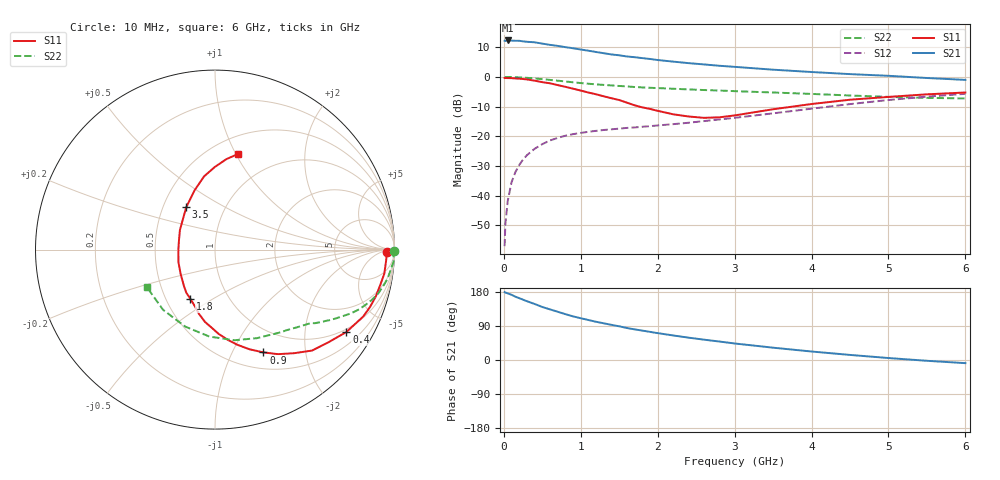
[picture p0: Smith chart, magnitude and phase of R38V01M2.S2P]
! SIEMENS Small Signal Semiconductors
! BFR181
! Si NPN RF Bipolar Junction Transistor in SOT23
! VCE = 8 V  IC = 1.2 mA
! Common Emitter S-Parameters:  May  1996
# GHz  S  MA  R  50
!  f  S11  S21  S12  S22
! GHz  MAG  ANG  MAG  ANG  MAG  ANG  MAG  ANG
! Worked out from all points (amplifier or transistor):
!   36 points, 10 MHz to 6 GHz, reference 50 ohm
!   highest |S21| = 12.3 dB at 50 MHz (marker M1)
!   |S21| within 3 dB of that: start of sweep to 987.8 MHz
!   unconditionally stable (mu >= 1): 1.967 GHz to 3.654 GHz
!   at 250 MHz: K = 0.17, MSG = 19.9 dB, |S12| = -27.9 dB
!   at 1.4 GHz: K = 0.80, MSG = 12.6 dB, |S12| = -17.7 dB
!   at 6 GHz: K = 0.86, MSG = 2.4 dB, |S12| = -5.7 dB
!   S11 on the Smith chart (normalised r, x): 10 MHz: 42, -14; 400 MHz: 0.90, -3.25; 900 MHz: 0.70, -1.33; 1.8 GHz: 0.66, -0.40; 3.5 GHz: 0.66, +0.34; 6 GHz: 0.67, +1.01
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0.01  0.9582 -0.8  4.069 179.2  0.0014 97.4  0.9984 -0.4
0.02  0.9573 -1.6  4.023 178.0  0.0033 92.5  0.9906 -0.8
0.05  0.9551 -3.9  4.115 175.9  0.008 87.2  0.9955 -2.0
0.1  0.9528 -8.1  4.088 172.1  0.0167 84.5  0.9968 -3.9
0.15  0.9415 -12.1  4.066 167.1  0.0248 81.3  0.9876 -5.9
0.2  0.9331 -16.3  4.062 163.2  0.0327 78.9  0.9808 -7.8
0.3  0.9061 -24.3  3.907 155.1  0.0479 75.0  0.9642 -11.4
0.4  0.8641 -32.1  3.832 147.9  0.0614 70.2  0.9432 -14.8
0.5  0.8153 -39.4  3.642 139.9  0.0735 66.1  0.9156 -18.0
0.6  0.7804 -46.1  3.47 133.6  0.0848 62.3  0.89 -20.5
0.7  0.7273 -52.5  3.33 127.3  0.0936 59.0  0.8632 -23.0
0.9  0.633 -64.8  3.04 115.1  0.1084 53.9  0.8111 -26.9
1.1  0.5446 -76.8  2.764 105.5  0.1188 50.6  0.7666 -30.3
1.4  0.4364 -92.3  2.39 92.7  0.1307 47.6  0.7185 -34.2
1.6  0.3679 -104.2  2.21 84.5  0.138 46.8  0.6914 -36.4
1.8  0.3065 -116.7  2.073 77.6  0.1443 47.5  0.6649 -38.4
2.2  0.2344 -144.9  1.81 64.8  0.1596 48.5  0.631 -43.2
2.8  0.2081 164.4  1.541 48.8  0.1913 51.2  0.5889 -51.4
3.5  0.2848 124.3  1.323 32.5  0.243 51.9  0.5459 -64.7
4.5  0.4124 98.5  1.114 13.4  0.3479 46.7  0.4858 -93.6
5.5  0.5082 82.8  0.958 -2.1  0.4645 34.8  0.4429 -130.8
6  0.5459 76.7  0.891 -8.3  0.5186 27.3  0.4332 -150.9
